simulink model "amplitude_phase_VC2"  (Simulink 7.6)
settings: Solver=ode45  StartTime=0.0  StopTime=10.0  RelTol=1e-3
InitFcn:
  | % Phase en rad du courant d'entrée
  | alpha=-30*pi/180;
  | % Amplitude du courant d'entrée
  | ampl=100;
undefined symbols (not defined in the file or in its folder): j

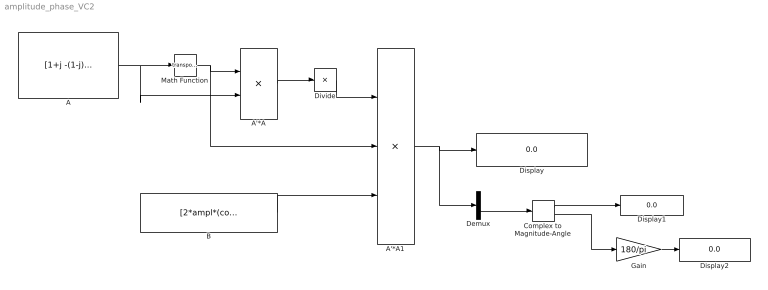
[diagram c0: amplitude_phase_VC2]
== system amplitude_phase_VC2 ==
  A : Constant  Value=[1+j -(1-j);1 -2/(1-j)]
  A'*A : Product  Multiplication=Matrix(*)
  A'*A1 : Product  Inputs=3  Multiplication=Matrix(*)
  B : Constant  Value=[2*ampl*(cos(alpha) +j*sin(alpha)); 0]
  Complex to Magnitude-Angle : ComplexToMagnitudeAngle
  Demux : Demux  Outputs=2
  Display : Display
  Display1 : Display
  Display2 : Display
  Divide : Product  Inputs=/  Multiplication=Matrix(*)
  Gain : Gain  Gain=180/pi
  Math Function : Math  Operator=transpose
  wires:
  A/1 -> Math Function/1, A'*A/2
  Math Function/1 -> A'*A/1, A'*A1/2
  A'*A/1 -> Divide/1
  Divide/1 -> A'*A1/1
  B/1 -> A'*A1/3
  A'*A1/1 -> Display/1, Demux/1
  Demux/2 -> Complex to Magnitude-Angle/1
  Complex to Magnitude-Angle/1 -> Display1/1
  Gain/1 -> Display2/1
  Complex to Magnitude-Angle/2 -> Gain/1
